PROGRAM MAIN_CM
VAR CONSTANT
	cInitFFT 		: ST_CM_ComplexFFT_InitPars := (nFFT_Length := cFFTLength, bForward := TRUE);															
END_VAR

VAR	
	fbComplexFFT	: FB_CMA_ComplexFFT :=(	stInitPars := cInitFFT, nOwnID := eID_FFT, aDestIDs := [eID_Sink] );														
	fbErrHist		: FB_HRErrHist; // error monitoring
END_VAR

// Call ComplexFFT 
fbComplexFFT.Call();
IF fbComplexFFT.bError THEN
	fbErrHist.AddError(bErr:=TRUE, hrErrCode:=fbComplexFFT.hrErrorCode, sErrSource:='MAIN_CM.fbComplexFFT'); // error monitoring
	// ToDo: if error
END_IF

END_PROGRAM
